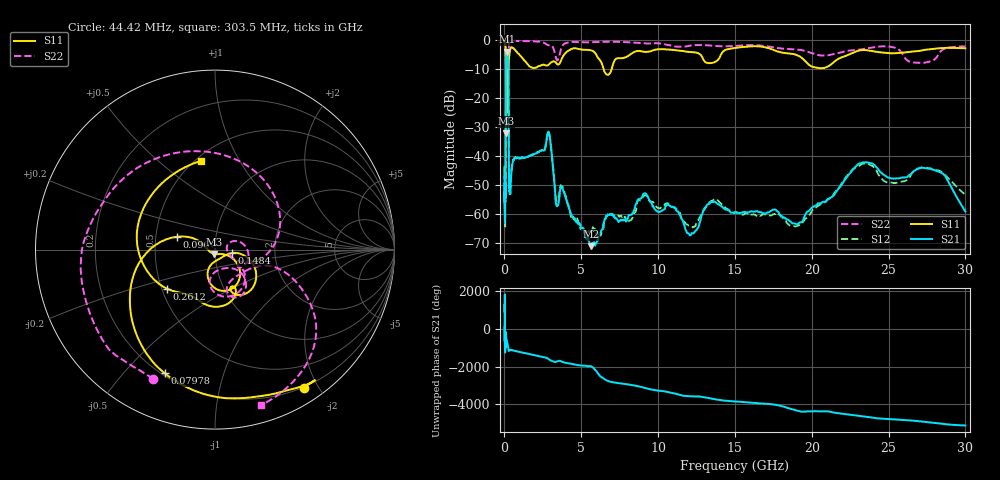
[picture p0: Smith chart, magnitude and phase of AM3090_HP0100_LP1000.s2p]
! Date/Time: Thu, Feb 28, 2019 1:57 PM
! Network Analyzer: Agilent Technologies E8364B Rev: A.07.50.67
! Sweep from 0.010 to 30.000 GHz, 1601 Points, Sweep Type: LOG
! Power Supply: 5.023 V, 0.002 A
# Hz S DB R 50
!freq MagS11 AngS11 MagS21 AngS21 MagS12 AngS12 MagS22 AngS22
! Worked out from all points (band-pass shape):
!   1601 points, 10 MHz to 30 GHz, reference 50 ohm
!   highest |S21| = -3.98 dB at 152.9 MHz (marker M1); lowest = -71.1 dB at 5.612 GHz (marker M2)
!   |S21| within 3 dB of the highest: 105.8 MHz to 239.3 MHz (133.5 MHz wide, 77.4 % of centre)
!   lowest |S11| = -32.2 dB at 104 MHz (marker M3), VSWR 1.05, Z = 49.5 - j2.4 ohm
!   |S11| at or under -10 dB: 94.41 MHz to 225.6 MHz (131.1 MHz wide, 82 % of centre); 231.5 MHz to 256.7 MHz (25.15 MHz wide, 10.3 % of centre); 6.455 GHz to 6.978 GHz (523.4 MHz wide, 7.79 % of centre)
!   |S22| runs from -23.6 to -0.1 dB; largest |S21 - S12| = 0.0099
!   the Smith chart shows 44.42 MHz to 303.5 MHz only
!   S11 on the Smith chart (normalised r, x): 44.42 MHz: 0.19, -1.82; 79.78 MHz: 0.21, -0.65; 96 MHz: 0.65, +0.10; 148.4 MHz: 1.21, -0.05; 261.2 MHz: 0.53, -0.26; 303.5 MHz: 0.53, +0.70
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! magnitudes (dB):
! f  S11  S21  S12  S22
! 10 MHz  -0.2  -47.8  -46.2  -0.7
! 38.04 MHz  -0.5  -59.4  -58.5  -1.5
! 44.42 MHz  -0.8  -57.9  -59.1  -2.0
! 79.78 MHz  -2.6  -48.2  -47.9  -4.8
! 96 MHz  -13.0  -14.9  -14.8  -11.6
! 104 MHz  -32.2  -7.6  -7.6  -23.2
! 119.6 MHz  -12.6  -5.1  -5.0  -15.8
! 144.7 MHz  -24.1  -4.0  -4.0  -16.0
! 148.4 MHz  -20.4  -4.0  -4.0  -15.7
! 152.9 MHz  -15.8  -4.0  -3.9  -14.8
! 261.2 MHz  -9.3  -15.2  -15.1  -9.8
! 303.5 MHz  -6.0  -50.7  -51.5  -0.9
! 550.5 MHz  -2.7  -41.9  -41.8  -0.2
! 2.084 GHz  -9.5  -39.1  -38.8  -0.5
! 2.884 GHz  -8.5  -31.8  -31.8  -1.8
! 3.402 GHz  -8.1  -57.3  -55.6  -6.9
! 5.612 GHz  -3.5  -71.1  -65.5  -0.8
! 7.926 GHz  -5.8  -62.5  -63.1  -0.7
! 9.027 GHz  -4.0  -53.2  -54.1  -1.1
! 19.03 GHz  -5.2  -63.6  -64.2  -3.3
! 23.48 GHz  -3.4  -42.2  -42.6  -3.0
! 30 GHz  -2.8  -59.2  -53.4  -2.2
